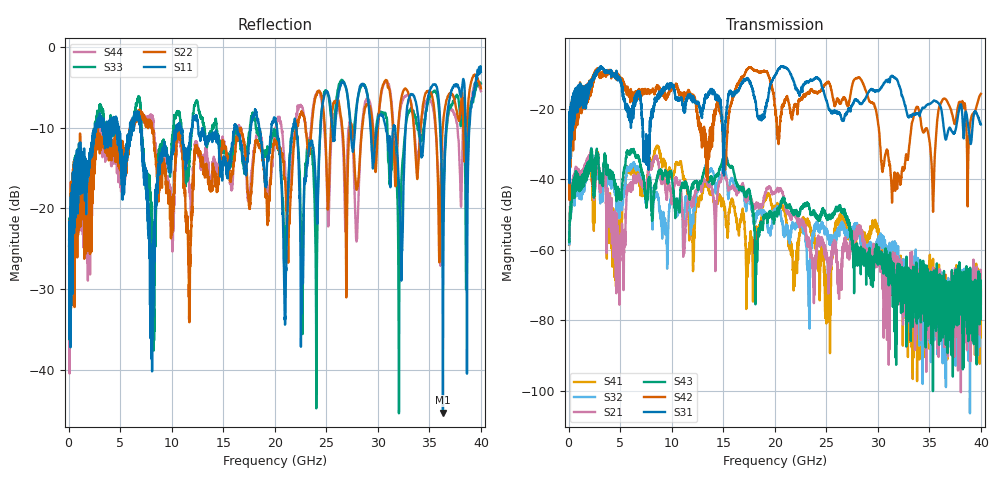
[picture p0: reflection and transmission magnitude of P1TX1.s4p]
!Agilent Technologies,N5245A,MY49151084,A.09.20.08
!Agilent N5245A: A.09.20.08
!Date: Thursday, March 01, 2012 14:30:53
!Correction: S11(Full 4 Port(1,2,3,4))
!S12(Full 4 Port(1,2,3,4))
!S13(Full 4 Port(1,2,3,4))
!S14(Full 4 Port(1,2,3,4))
!S21(Full 4 Port(1,2,3,4))
!S22(Full 4 Port(1,2,3,4))
!S23(Full 4 Port(1,2,3,4))
!S24(Full 4 Port(1,2,3,4))
!S31(Full 4 Port(1,2,3,4))
!S32(Full 4 Port(1,2,3,4))
!S33(Full 4 Port(1,2,3,4))
!S34(Full 4 Port(1,2,3,4))
!S41(Full 4 Port(1,2,3,4))
!S42(Full 4 Port(1,2,3,4))
!S43(Full 4 Port(1,2,3,4))
!S44(Full 4 Port(1,2,3,4))
!S4P File: Measurements: <S11,S12,S13,S14>,
!<S21,S22,S23,S24>,
!<S31,S32,S33,S34>,
!<S41,S42,S43,S44>:
# Hz S  dB  R 50
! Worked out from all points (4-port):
!   3996 points, 50 MHz to 40 GHz, reference 50 ohm
!   strongest paths, dB at 50 MHz, 10.04 GHz, 20.03 GHz, 30.02 GHz, 40 GHz:
!     S31: -23.6, -13.6, -10.6, -15.0, -24.4
!     S42: -25.5, -13.5, -19.1, -24.0, -15.8
!     S43: -57.2, -40.0, -49.3, -59.6, -72.0
!     S21: -57.5, -46.8, -43.6, -59.7, -75.2
!     S32: -54.8, -44.7, -49.7, -58.6, -79.0
!     S41: -58.6, -39.8, -48.1, -54.2, -71.4
!   lowest |S11| = -45.3 dB at 36.32 GHz (marker M1), VSWR 1.01, Z = 49.5 + j0.219 ohm
!   |S11| at or under -10 dB: start of sweep to 2.585 GHz; 7.013 GHz to 10.45 GHz (3.439 GHz wide, 39.4 % of centre); 12.58 GHz to 16.08 GHz (3.504 GHz wide, 24.5 % of centre)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
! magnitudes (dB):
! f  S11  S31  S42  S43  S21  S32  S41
! 50 MHz  -23.9  -23.6  -25.5  -57.2  -57.5  -54.8  -58.6
! 15.18 GHz  -14.5  -26.5  -37.3  -33.3  -38.9  -37.0  -48.2
! 17.53 GHz  -12.0  -11.9  -8.2  -43.2  -45.7  -45.3  -58.0
! 28.26 GHz  -4.9  -18.3  -11.3  -64.3  -54.9  -56.0  -53.7
! 31.52 GHz  -9.8  -11.0  -40.6  -63.8  -64.1  -59.9  -73.1
! 36.32 GHz  -45.3  -23.4  -17.3  -69.6  -78.0  -85.3  -67.7
! 40 GHz  -3.1  -24.4  -15.8  -72.0  -75.2  -79.0  -71.4
